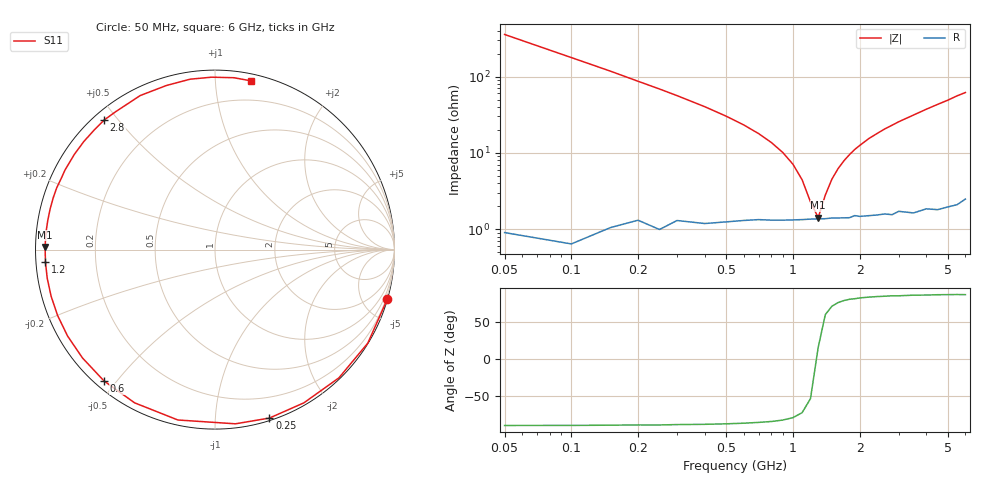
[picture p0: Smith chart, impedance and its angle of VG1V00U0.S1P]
! Infineon Technologies  Discrete & RF Semiconductors
! BB 831
! Si Tuning Diode in SOD323
! VR = 1 V
! S-Parameters:  July  1999
# GHz  S  MA  R  50
!  f  S11
! GHz  MAG  ANG
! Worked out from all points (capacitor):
!   34 points, 50 MHz to 6 GHz, reference 50 ohm
!   read as one part to ground: C = 8.92 pF near 50 MHz
!   lowest |Z| = 1.42 ohm at 1.3 GHz (marker M1)
!   series resonance near 1.282 GHz, so ESL is about 1.7 nH
!   S11 on the Smith chart (normalised r, x): 50 MHz: 0.02, -7.12; 250 MHz: 0.02, -1.37; 600 MHz: 0.03, -0.46; 1.2 GHz: 0.03, -0.04; 2.8 GHz: 0.03, +0.46; 6 GHz: 0.05, +1.23
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0.05  0.9993 -16.0
0.1  0.9981 -31.5
0.15  0.9936 -46.0
0.2  0.987 -59.9
0.25  0.9863 -72.1
0.3  0.9773 -83.3
0.4  0.9716 -102.3
0.5  0.9641 -117.7
0.6  0.958 -130.2
0.7  0.9537 -140.7
0.8  0.9522 -149.6
0.9  0.9507 -157.3
1  0.9493 -164.1
1.2  0.9472 -175.8
1.3  0.9468 179.1
1.4  0.9466 174.4
1.6  0.9461 166.1
1.9  0.944 155.2
2.2  0.9464 145.9
2.4  0.947 140.5
2.8  0.9501 130.6
3  0.947 125.9
3.5  0.9541 115.9
4  0.9536 106.5
4.5  0.9595 98.3
5  0.9608 91.1
5.5  0.9634 83.7
6  0.9614 78.0
